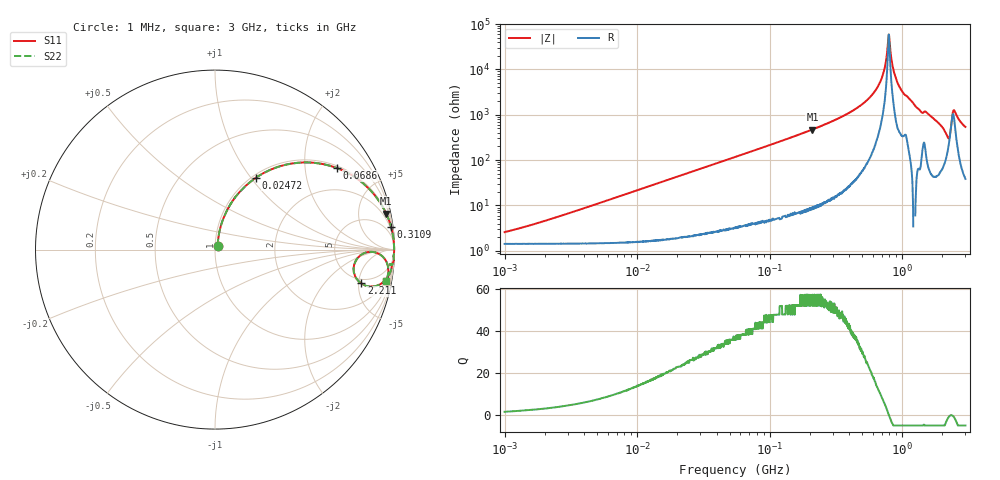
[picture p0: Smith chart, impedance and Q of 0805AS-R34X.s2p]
!s-Parameter Generated by FASTRON Sdn. Bhd.
!FASTRON P/N : 0805AS-R34X
!Keysight Technologies: E4991B_MY54100416_A.01.15
!Date: Mon Jun 15 12:54:24 2026
!Version  :Rev01  Mon Jun 15 12:54:24 2026
!Data & Calibration Information:
!Freq  S11  S21  S12  S22
!PortZ  Port1:50+j0  Port2:50+j0
!When reading reference impedance value at option line is always used.
! Remarks : This data is being provided solely for informational purposes.
# Hz S dB R 50
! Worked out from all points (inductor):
!   1601 points, 1 MHz to 3 GHz, reference 50 ohm
!   read as one part in series: L = 344 nH near 1.985 MHz
!   highest Q = 57.1 at 210.5 MHz (marker M1), where L = 357 nH
!   self-resonance near 792.6 MHz
!   S11 on the Smith chart (normalised r, x): 1 MHz: 1.03, +0.04; 24.72 MHz: 1.04, +1.06; 68.6 MHz: 1.07, +2.93; 310.9 MHz: 1, +15; 2.211 GHz: 4.31, -5.41; 3 GHz: 2, -11
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1000000  -31.90 55.5  -0.12 -1.2  -0.12 -1.2  -31.90 55.5
3804036  -21.70 75.4  -0.15 -4.6  -0.15 -4.6  -21.70 75.4
1.447069e7  -10.70 69.9  -0.54 -17.0  -0.54 -17.0  -10.70 69.9
2.471848e7  -6.72 60.3  -1.22 -27.4  -1.22 -27.4  -6.72 60.3
5.504702e7  -2.48 39.7  -3.88 -48.7  -3.88 -48.7  -2.48 39.7
6.860483e7  -1.76 33.9  -5.08 -54.7  -5.08 -54.7  -1.76 33.9
2.083556e8  -0.23 12.0  -13.60 -76.9  -13.60 -76.9  -0.23 12.0
2.104513e8  -0.22 11.9  -13.70 -77.1  -13.70 -77.1  -0.22 11.9
3.10929e8  -0.10 7.4  -17.80 -81.4  -17.80 -81.4  -0.10 7.4
4.781416e8  -0.04 3.7  -23.90 -84.5  -23.90 -84.5  -0.04 3.7
6.171487e8  -0.02 1.8  -30.10 -84.8  -30.10 -84.8  -0.02 1.8
7.099691e8  -0.02 0.8  -37.00 -81.8  -37.00 -81.8  -0.02 0.8
7.730077e8  -0.01 0.2  -48.60 -63.0  -48.60 -63.0  -0.01 0.2
7.925923e8  -0.01 0.0  -55.40 -4.4  -55.40 -4.4  -0.01 0.0
8.12673e8  -0.02 -0.2  -49.00 59.9  -49.00 59.9  -0.02 -0.2
8.848309e8  -0.02 -0.8  -37.10 81.5  -37.10 81.5  -0.02 -0.8
1.002744e9  -0.03 -1.8  -30.20 82.2  -30.20 82.2  -0.03 -1.8
1.367504e9  -0.07 -4.6  -21.80 82.3  -21.80 82.3  -0.07 -4.6
1.874306e9  -0.19 -8.5  -16.60 77.5  -16.60 77.5  -0.19 -8.5
2.210833e9  -1.55 -13.0  -11.60 45.6  -11.60 45.6  -1.55 -13.0
2.468121e9  -0.45 -3.3  -22.40 46.5  -22.40 46.5  -0.45 -3.3
3e9  -0.26 -10.4  -14.90 75.5  -14.90 75.5  -0.26 -10.4
